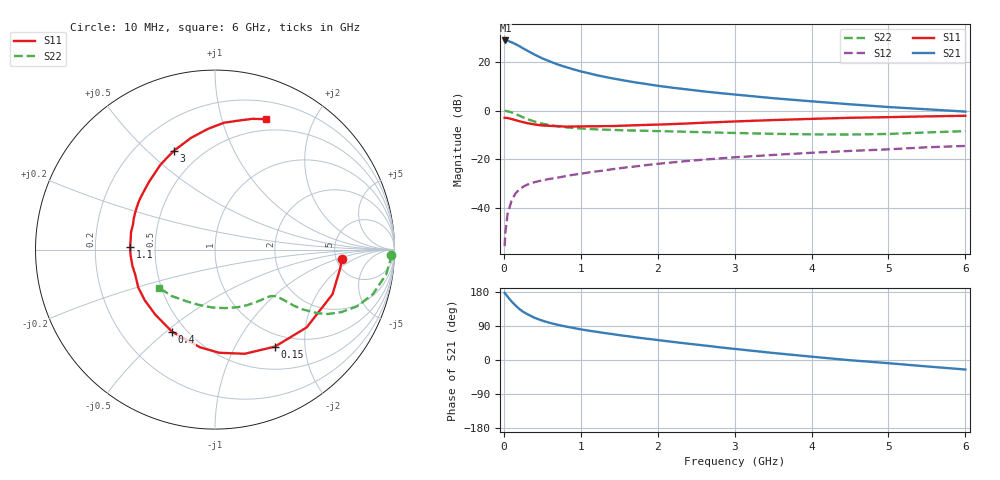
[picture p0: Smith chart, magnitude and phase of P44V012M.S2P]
! SIEMENS Small Signal Semiconductors
! BFP182
! Si NPN RF Bipolar Junction Transistor in SOT143
! VCE = 4 V  IC = 12 mA
! Common Emitter S-Parameters:  March  1996
# GHz  S  MA  R  50
!  f  S11  S21  S12  S22
! GHz  MAG  ANG  MAG  ANG  MAG  ANG  MAG  ANG
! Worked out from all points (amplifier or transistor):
!   36 points, 10 MHz to 6 GHz, reference 50 ohm
!   highest |S21| = 28.9 dB at 20 MHz (marker M1)
!   |S21| within 3 dB of that: start of sweep to 237.1 MHz
!   unconditionally stable (mu >= 1): 1.112 GHz to 5.366 GHz
!   at 250 MHz: K = 0.36, MSG = 28.5 dB, |S12| = -31.4 dB
!   at 1.4 GHz: K = 1.09, MAG = 17.0 dB, |S12| = -24.2 dB
!   at 6 GHz: K = 0.93, MSG = 7.1 dB, |S12| = -14.6 dB
!   S11 on the Smith chart (normalised r, x): 10 MHz: 5.59, -1.19; 150 MHz: 0.81, -1.47; 400 MHz: 0.42, -0.52; 1.1 GHz: 0.36, +0.01; 3 GHz: 0.36, +0.60; 6 GHz: 0.38, +1.39
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0.01  0.7081 -4.3  27.8 177.2  0.0016 81.6  0.9788 -1.6
0.02  0.7059 -8.3  27.82 174.9  0.0031 82.6  0.9798 -3.3
0.05  0.7004 -20.8  27.34 166.8  0.0076 83.7  0.9634 -8.3
0.1  0.6699 -40.3  25.57 154.8  0.0138 71.1  0.9138 -15.8
0.15  0.6354 -58.3  23.48 144.2  0.0195 64.2  0.8518 -21.8
0.2  0.6035 -74.1  21.36 134.9  0.0234 59.3  0.7855 -26.3
0.25  0.5753 -87.6  19.15 127.4  0.0268 54.8  0.7244 -29.7
0.3  0.5509 -98.7  17.33 121.6  0.0294 51.6  0.6721 -31.8
0.4  0.5164 -117.6  14.2 111.4  0.0334 48.7  0.5917 -34.3
0.5  0.4917 -132.7  11.89 103.8  0.0364 46.6  0.5364 -35.5
0.6  0.4826 -144.0  10.26 97.9  0.0391 46.1  0.4975 -35.9
0.7  0.4769 -153.7  8.89 92.9  0.0414 45.9  0.4715 -36.3
0.9  0.4691 -168.9  7.102 84.8  0.0474 46.4  0.4368 -37.0
1.1  0.4737 178.5  5.883 77.5  0.0529 47.1  0.417 -38.4
1.5  0.4842 159.3  4.34 65.6  0.0643 47.5  0.3948 -42.3
1.8  0.5021 147.7  3.619 57.6  0.0732 46.8  0.3837 -46.2
2.2  0.5262 134.6  2.945 47.7  0.0855 45.0  0.3713 -52.6
3  0.5955 112.8  2.138 29.3  0.1086 39.6  0.3452 -68.4
3.5  0.6359 102.3  1.796 18.6  0.1215 35.8  0.331 -80.0
4.5  0.7083 86.0  1.344 -0.6  0.147 28.0  0.3207 -106.4
5.5  0.7575 74.1  1.06 -17.0  0.1748 20.5  0.3536 -133.0
6  0.7798 68.8  0.951 -25.1  0.1863 15.8  0.3767 -145.7
